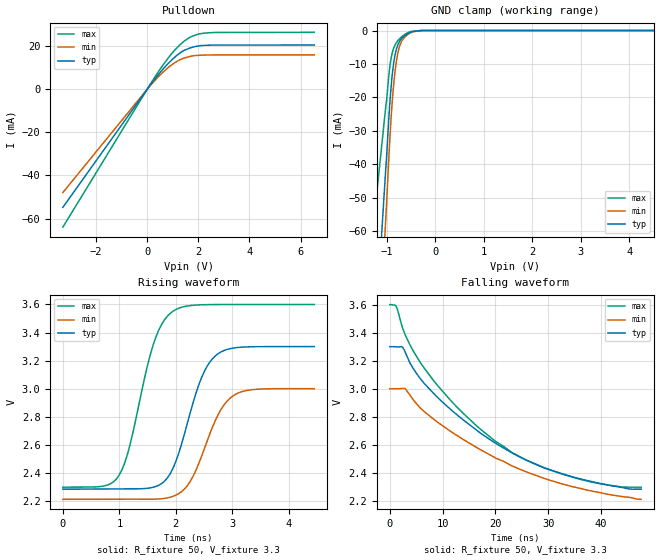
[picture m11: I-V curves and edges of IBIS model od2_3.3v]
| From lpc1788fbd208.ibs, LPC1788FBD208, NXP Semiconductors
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[Model]   od2_3.3v
Model_type I/O_open_drain
Vinl=9.900E-01
Vinh=2.310E+00
Vref=3.300E+00
Rref=2.000E+03
Cref=0.000E+00
Vmeas=1.650E+00
C_comp   5.160E-13   4.910E-13   5.420E-13
[Voltage Range]   3.300E+00   3.000E+00   3.600E+00
[POWER Clamp Reference]   3.300E+00   3.000E+00   3.600E+00
[GND Clamp Reference]   0.000E+00   0.000E+00   0.000E+00
[Pullup Reference]   3.300E+00   3.000E+00   3.600E+00
[Pulldown Reference]   0.000E+00   0.000E+00   0.000E+00
[Temperature Range]   25   85   -40
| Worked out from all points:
|   slope of the pulldown table from 0 to 0.495 V, typ, clamps not added: 64.9 ohm
|   GND clamp passes 1 mA (typ) near -0.57 V on its own axis
|   rising waveform, R_fixture 50, V_fixture 3.3: 20-80 % time 470ps typ, 490ps min, 462ps max; typ from 2.28 V to 3.3 V
|   falling waveform, R_fixture 50, V_fixture 3.3: 20-80 % time 20.8ns typ, 22.3ns min, 19.2ns max; typ from 3.3 V to 2.28 V
[GND Clamp]
-3.3V     -568mA     -692.7mA   -341mA
-1.025V   -41.76mA   -56.76mA   -23.04mA
-964.7mV  -27.52mA   -39.73mA   -14.26mA
-924.8mV  -18.98mA   -29.09mA   -9.42mA
-884.9mV  -12.65mA   -20.46mA   -6.462mA
-825mV    -6.857mA   -11.43mA   -4.158mA
-785.1mV  -4.764mA   -7.603mA   -3.283mA
-725.2mV  -2.935mA   -4.187mA   -2.28mA
-645.4mV  -1.707mA   -2.177mA   -1.314mA
-525.6mV  -616.5uA   -810.9uA   -398.4uA
-266.1mV  0A         0A         0A
6.6V      0A         0A         0A
[Pulldown]
-3.3V     -54.79mA   -47.91mA   -63.96mA
153mV     2.489mA    2.147mA    2.94mA
512.3mV   7.874mA    6.706mA    9.412mA
891.5mV   12.77mA    10.7mA     15.54mA
1.131V    15.41mA    12.66mA    18.82mA
1.43V     17.91mA    14.39mA    22.12mA
1.77V     19.45mA    15.47mA    24.58mA
2.269V    20.35mA    15.84mA    26.06mA
6.54V     20.51mA    15.9mA     26.38mA
[Rising Waveform]
R_fixture = 50
V_fixture = 3.3
V_fixture_min = 3
V_fixture_max = 3.6
0s        2.284V     2.211V     2.298V
1ns       2.285V     2.212V     2.386V
1.2ns     2.286V     2.212V     2.619V
1.6ns     2.297V     2.212V     3.314V
1.95ns    2.433V     2.233V     3.552V
2.3ns     2.893V     2.372V     3.594V
2.5ns     3.12V      2.567V     3.598V
2.7ns     3.234V     2.774V     3.6V
3.15ns    3.295V     2.976V     3.6V
4.45ns    3.3V       3V         3.6V
[Falling Waveform]
R_fixture = 50
V_fixture = 3.3
V_fixture_min = 3
V_fixture_max = 3.6
0s        3.3V       3V         3.6V
1.199ns   3.299V     3V         3.589V
2.447ns   3.295V     3.003V     3.433V
5.194ns   3.102V     2.888V     3.223V
8.241ns   2.969V     2.785V     3.061V
13.99ns   2.776V     2.636V     2.822V
20.13ns   2.609V     2.504V     2.622V
25.82ns   2.491V     2.407V     2.491V
32.62ns   2.394V     2.321V     2.392V
47.6ns    2.284V     2.211V     2.298V
[Ramp]
dV/dt_r   6.0988E-01/4.6880E-10   4.7340E-01/4.8990E-10   7.8133E-01/4.6000E-10
dV/dt_f   6.0988E-01/2.0795E-08   4.7340E-01/2.2268E-08   7.8133E-01/1.9147E-08
R_load = 50
